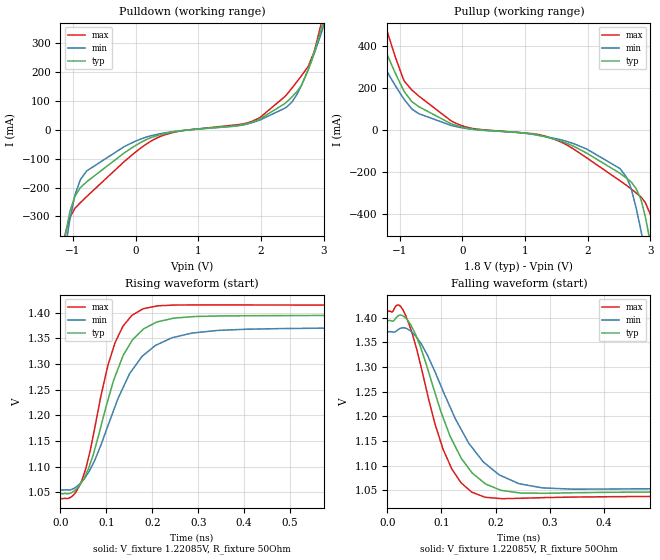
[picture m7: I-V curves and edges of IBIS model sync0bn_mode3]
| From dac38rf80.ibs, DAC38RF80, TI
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|   sync0bn_mode3 Model
[Model]   sync0bn_mode3
Model_type   Output
Polarity   Non-Inverting
Vmeas = 1.220854
Vref = 1.220854
Cref = 2pF
Rref = 200
|   typ   min   max
|   (nom PVT)   (fast PVT)   (slow PVT)
C_comp   6.288e-13   6.288e-13   7.537e-13
| Where nom  PVT is Nominal Process, 1.8V, 27C
|   Fast PVT is Strong Process,  1.89V, -40C
|   Slow PVT is Weak Process,   1.71V, 105C
[Voltage Range]   1.8   1.71   1.89
|Junction Temperature
[Temperature Range]   27   105   -40
[Pullup Reference]   1.8   1.71   1.89
[Pulldown Reference]   0   0   0
[Power Clamp Reference]   1.8   1.71   1.89
[GND Clamp Reference]   0   0   0
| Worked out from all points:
|   slope of the pulldown table from 0 to 0.27 V, typ, clamps not added: 9.38 ohm
|   slope of the pullup table from 0 to 0.27 V, typ, clamps not added: 21.4 ohm
|   falling waveform, V_fixture 1.22085V, R_fixture 50Ohm: 20-80 % time 69.4ps typ, 88.9ps min, 57.3ps max; typ from 1.39 V to 1.05 V
|   rising waveform, V_fixture 1.22085V, R_fixture 50Ohm: 20-80 % time 73ps typ, 95ps min, 57.8ps max; typ from 1.05 V to 1.39 V
[Pulldown]
|   Voltage   I(typ)   I(min)   I(max)
-1.8V     -1.509A    -1.416A    -1.673A
-1.114V   -354.6mA   -397.5mA   -352.7mA
-972.2mV  -232mA     -229.2mA   -272.6mA
-780.8mV  -180mA     -142.5mA   -231mA
-31.86mV  -58.73mA   -42.6mA    -82.69mA
570.1mV   -9.136mA   -7.65mA    -11.16mA
1.838V    24.87mA    23.13mA    27.29mA
2.389V    91.4mA     75.19mA    115.8mA
2.646V    152.5mA    152.6mA    186.1mA
2.757V    208.4mA    208.8mA    219.4mA
2.97V     353.2mA    338.4mA    374.3mA
3.6V      958.1mA    1.326A     1.097A
[Pullup]
|   Voltage   I(typ)   I(min)   I(max)
-1.8V     891.5mA    1.047A     1.127A
-1.513V   590.8mA    475.5mA    776.8mA
-1.166V   332.3mA    256.8mA    433.5mA
-927mV    180.1mA    142.5mA    230.1mA
-698.4mV  109.6mA    76.23mA    160.1mA
-4.5mV    12.63mA    8.919mA    18.69mA
1.976V    -110.4mA   -91.07mA   -132.6mA
2.619V    -230.3mA   -226.1mA   -265mA
2.857V    -340.5mA   -491.5mA   -322.8mA
2.993V    -529.5mA   -693.1mA   -399.8mA
3.069V    -657.8mA   -804.8mA   -490.7mA
3.6V      -1.566A    -1.597A    -1.554A
[Ramp]
R_load = 50
|   typ   min   max
dV/dt_r   0.151524/9.35226e-11   0.153496/1.25759e-10   0.168668/6.55076e-11
dV/dt_f   0.207904/6.93701e-11   0.189967/8.88847e-11   0.224938/5.72723e-11
[Falling Waveform]
V_fixture = 1.22085V
V_fixture_min = 1.21326V
V_fixture_max = 1.22554V
R_fixture = 50Ohm
|   Time   V(typ)   V(min)   V(max)
0s        1.394V     1.371V     1.413V
21.21ps   1.405V     1.377V     1.426V
33.73ps   1.399V     1.379V     1.405V
62.31ps   1.337V     1.348V     1.3V
88.01ps   1.248V     1.29V      1.184V
119.1ps   1.153V     1.211V     1.093V
156.9ps   1.085V     1.136V     1.046V
211.7ps   1.049V     1.079V     1.033V
341.8ps   1.045V     1.052V     1.036V
5ns       1.048V     1.055V     1.038V
[Rising Waveform]
V_fixture = 1.22085V
V_fixture_min = 1.21326V
V_fixture_max = 1.22554V
R_fixture = 50Ohm
|   Time   V(typ)   V(min)   V(max)
0s        1.048V     1.055V     1.038V
24.3ps    1.05V      1.056V     1.042V
47.21ps   1.071V     1.072V     1.075V
71.24ps   1.123V     1.106V     1.16V
103.2ps   1.229V     1.179V     1.297V
136.1ps   1.316V     1.254V     1.374V
211.7ps   1.382V     1.338V     1.413V
341.8ps   1.393V     1.365V     1.415V
574.2ps   1.394V     1.37V      1.415V
5ns       1.394V     1.372V     1.413V
